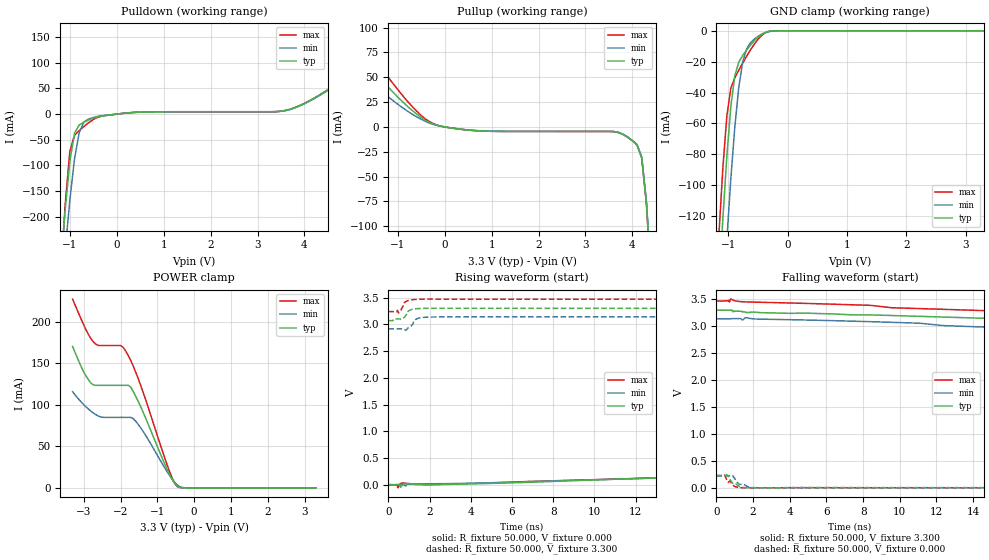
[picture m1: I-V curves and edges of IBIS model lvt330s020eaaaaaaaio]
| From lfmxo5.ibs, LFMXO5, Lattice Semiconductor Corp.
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[Model] lvt330s020eaaaaaaaio
Model_type I/O
Polarity   Non-Inverting
Enable   Active-Low
Vinl =  0.800V
Vinh =  2.000V
Vmeas =  1.650V
Cref =  0.0F
Rref =  1.000M
Vref =  0.0V
C_comp   5.000pF   4.000pF   5.500pF
[Temperature Range]   25.000   0.125k   -40.000
[Voltage Range]   3.300V   3.140V   3.470V
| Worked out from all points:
|   slope of the pulldown table from 0 to 0.495 V, typ, clamps not added: 128 ohm
|   slope of the pullup table from 0 to 0.495 V, typ, clamps not added: 158 ohm
|   GND clamp passes 1 mA (typ) near -0.37 V on its own axis
|   POWER clamp passes 1 mA (typ) near -0.42 V on its own axis
|   rising waveform, R_fixture 50.000, V_fixture 0.000: 20-80 % time 10.4ns typ, 11.2ns min, 10.8ns max; typ from 0.001 V to 0.227 V
|   rising waveform, R_fixture 50.000, V_fixture 3.300: 20-80 % time 288ps typ, 269ps min, 201ps max; typ from 3.07 V to 3.3 V
|   falling waveform, R_fixture 50.000, V_fixture 3.300: 20-80 % time 15.4ns typ, 9.07ns min, 10.1ns max; typ from 3.3 V to 3.07 V
|   falling waveform, R_fixture 50.000, V_fixture 0.000: 20-80 % time 442ps typ, 586ps min, 391ps max; typ from 0.227 V to 0.001 V
[GND_clamp]
|Voltage   I(typ)   I(min)   I(max)
-3.3V     -1.887A    -1.873A    -1.902A
-1.156V   -166.9mA   -224mA     -132.1mA
-1.089V   -121.5mA   -178.4mA   -88.64mA
-1.022V   -81.05mA   -135.2mA   -54.94mA
-955mV    -48.98mA   -95.79mA   -37.15mA
-888mV    -28.98mA   -62.05mA   -30.42mA
-821mV    -20.23mA   -36.35mA   -25.49mA
-754mV    -15.89mA   -19.89mA   -20.81mA
-687mV    -12.34mA   -11.44mA   -16.31mA
-620mV    -9.094mA   -7.515mA   -12.09mA
-419mV    -1.869mA   -1.836mA   -2.383mA
3.3V      0A         0A         0A
[POWER_clamp]
|Voltage   I(typ)   I(min)   I(max)
-3.3V     170.3mA    115.9mA    227.4mA
-2.998V   139.6mA    100.3mA    196.3mA
-2.797V   125.9mA    92.2mA     179.4mA
-2.596V   123.5mA    86.45mA    171.5mA
-1.993V   123.5mA    84.93mA    171.5mA
-1.792V   123.5mA    84.93mA    159.6mA
-1.658V   116.4mA    83.68mA    147.1mA
-1.457V   98.28mA    72.65mA    124.1mA
-720mV    21.08mA    18.41mA    25.96mA
-452mV    1.573mA    3.148mA    1.229mA
-184mV    5.589uA    37.85uA    1.612uA
3.3V      0A         0A         0A
[Pulldown]
|Voltage   I(typ)   I(min)   I(max)
-3.3V     -3.023A    -2.882A    -4.076A
-1.2V     -299.4mA   -373.4mA   -326mA
-1.1V     -186.9mA   -266.3mA   -176.8mA
-1V       -92.5mA    -167.9mA   -72.23mA
-900mV    -37.01mA   -86.9mA    -41.16mA
-800mV    -21.11mA   -36.05mA   -32.24mA
-600mV    -11.54mA   -9.523mA   -16.85mA
300mV     2.818mA    2.733mA    2.818mA
3.7V      9.422mA    9.139mA    9.422mA
5.3V      93.3mA     90.5mA     93.3mA
6.1V      115.6mA    112.2mA    115.6mA
6.6V      168.3mA    163.3mA    168.3mA
[Pullup]
|Voltage   I(typ)   I(min)   I(max)
-3.3V     139.8mA    86.3mA     180mA
-2.9V     101.3mA    74.5mA     141.2mA
-2.7V     91.2mA     69.71mA    121.2mA
-2V       78.6mA     57.94mA    97.4mA
-800mV    21.01mA    16.14mA    26.23mA
-200mV    2.224mA    1.901mA    2.518mA
3.8V      -7.525mA   -7.299mA   -7.525mA
4.1V      -18.2mA    -17.66mA   -18.2mA
4.2V      -31.31mA   -30.37mA   -31.31mA
4.3V      -77.3mA    -75mA      -77.3mA
4.4V      -155.6mA   -151mA     -155.6mA
6.6V      -2.513A    -2.438A    -2.513A
[Ramp]
| variable   typ   min   max
dV/dt_r   0.136/10.320n   0.131/11.213n   0.136/10.796n
dV/dt_f   0.138/10.696n   0.134/10.128n   0.139/11.426n
R_load = 50.000
[Rising Waveform]
R_fixture = 50.000
V_fixture = 0.000
V_fixture_min = 0.000
V_fixture_max = 0.000
|  time   V(typ)   V(min)   V(max)
0s        974.6uV    2.777mV    974.6uV
395ps     1.025mV    2.399mV    3.382mV
474ps     1.149mV    2.686mV    -57.42mV
546ps     2.654mV    2.824mV    8.255mV
605ps     -44.68mV   2.886mV    25.48mV
693ps     6.203mV    2.778mV    33.22mV
823ps     20.17mV    -23.42mV   29.09mV
942ps     24.73mV    12.75mV    21.29mV
2.297ns   4.707mV    19.74mV    6.25mV
20ns      227.4mV    220.6mV    227.5mV
[Rising Waveform]
R_fixture = 50.000
V_fixture = 3.300
V_fixture_min = 3.140
V_fixture_max = 3.470
|  time   V(typ)   V(min)   V(max)
0s        3.069V     2.916V     3.239V
438ps     3.102V     2.916V     3.261V
507ps     3.101V     2.917V     3.215V
631ps     3.093V     2.917V     3.282V
743ps     3.125V     2.917V     3.391V
852ps     3.169V     2.891V     3.428V
1.051ns   3.267V     2.957V     3.454V
1.292ns   3.29V      3.082V     3.466V
1.547ns   3.297V     3.123V     3.47V
20ns      3.3V       3.14V      3.47V
[Falling Waveform]
R_fixture = 50.000
V_fixture = 3.300
V_fixture_min = 3.140
V_fixture_max = 3.470
|  time   V(typ)   V(min)   V(max)
0s        3.3V       3.14V      3.47V
671ps     3.301V     3.141V     3.481V
721ps     3.3V       3.141V     3.455V
802ps     3.3V       3.142V     3.506V
1.429ns   3.268V     3.118V     3.458V
1.599ns   3.258V     3.16V      3.455V
11.09ns   3.186V     3.058V     3.33V
16.15ns   3.143V     2.967V     3.276V
19.23ns   3.108V     2.926V     3.245V
20ns      3.069V     2.916V     3.239V
[Falling Waveform]
R_fixture = 50.000
V_fixture = 0.000
V_fixture_min = 0.000
V_fixture_max = 0.000
|  time   V(typ)   V(min)   V(max)
0s        227.4mV    220.6mV    227.5mV
433ps     227.1mV    220.3mV    239.4mV
597ps     238.4mV    220mV      130.3mV
649ps     219.5mV    220.4mV    100.8mV
749ps     158.1mV    228.3mV    128.3mV
852ps     98.65mV    234.8mV    72.34mV
1.239ns   26.73mV    66.64mV    4.887mV
1.421ns   8.236mV    62.65mV    766.3uV
2.261ns   -477.7uV   823.2uV    -880.9uV
20ns      974.6uV    2.777mV    974.6uV
